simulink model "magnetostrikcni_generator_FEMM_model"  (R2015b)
settings: Solver=VariableStepAuto  StartTime=0.0  StopTime=1  FixedStep=1e-3  RelTol=1e-3
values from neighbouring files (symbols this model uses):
  A = (pi*d_terf^2)/4    (= 5.02654824574e-05)    [parametry_magneto.m]    (also in P_016_80_parametry.m = 0.00020106192983)
  delta_x = 4e-4    (= 0.0004)    [parametry_magneto.m]    (also in piezoelektricky_genarator_parametry.m)
  k_amp = F_in/delta_x    (= 6821500)    [parametry_magneto.m]    (also in piezoelektricky_genarator_parametry.m)
  L = (perm*(N_c^2)*A_c)/l_c    [parametry_magneto.m]
  N_c = N_c_row*floor(N_c/N_c_row)    [parametry_magneto.m]
  p = polyfit(napeti,fi,3)    [parametry_magneto.m]
  Rc = 4*(ro_Cu*l_d)/(pi*d_d^2)    [parametry_magneto.m]
  Rz = 250    [parametry_magneto.m]

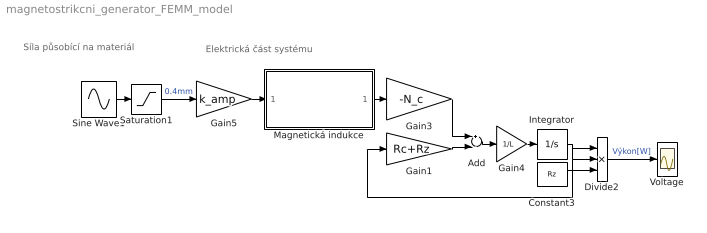
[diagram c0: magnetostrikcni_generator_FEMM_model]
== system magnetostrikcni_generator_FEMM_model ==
  note: Elektrická část systému
  note: Síla působící na materiál
  Add : Sum  Inputs=+-
  Constant3 : Constant  Value=Rz
  Divide2 : Product  Inputs=***
  Gain1 : Gain  Gain=Rc+Rz
  Gain3 : Gain  Gain=-N_c
  Gain4 : Gain  Gain=1/L
  Gain5 : Gain  Gain=k_amp
  Integrator : Integrator
  Magnetická indukce : Subsystem
  Saturation1 : Saturate  UpperLimit=delta_x  LowerLimit=0
  Sine Wave1 : Sin  Amplitude=2*delta_x  Frequency=2*pi*2  SampleTime=0
  Voltage : Scope
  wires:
  Sine Wave1/1 -> Saturation1/1
  Gain3/1 -> Add/1
  Add/1 -> Gain4/1
  Gain1/1 -> Add/2
  Gain4/1 -> Integrator/1
  Integrator/1 -> Divide2/1, Divide2/2, Gain1/1
  Constant3/1 -> Divide2/3
  Divide2/1 -> Voltage/1  "Výkon[W]"
  Magnetická indukce/1("derivace ") -> Gain3/1
  Saturation1/1 -> Gain5/1  "0.4mm"
  Gain5/1 -> Magnetická indukce/1(Síla na Stack)

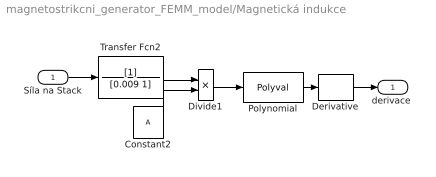
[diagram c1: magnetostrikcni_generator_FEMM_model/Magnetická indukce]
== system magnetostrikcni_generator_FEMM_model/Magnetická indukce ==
  Síla na Stack : Inport
  Constant2 : Constant  Value=A
  Derivative : Derivative
  Divide1 : Product  Inputs=*/
  Polynomial : Polyval  Coefs=p
  Transfer Fcn2 : TransferFcn  Denominator=[0.009 1]
  "derivace " : Outport
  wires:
  Constant2/1 -> Divide1/2
  Síla na Stack/1 -> Transfer Fcn2/1
  Divide1/1 -> Polynomial/1
  Polynomial/1 -> Derivative/1
  Derivative/1 -> "derivace "/1
  Transfer Fcn2/1 -> Divide1/1
